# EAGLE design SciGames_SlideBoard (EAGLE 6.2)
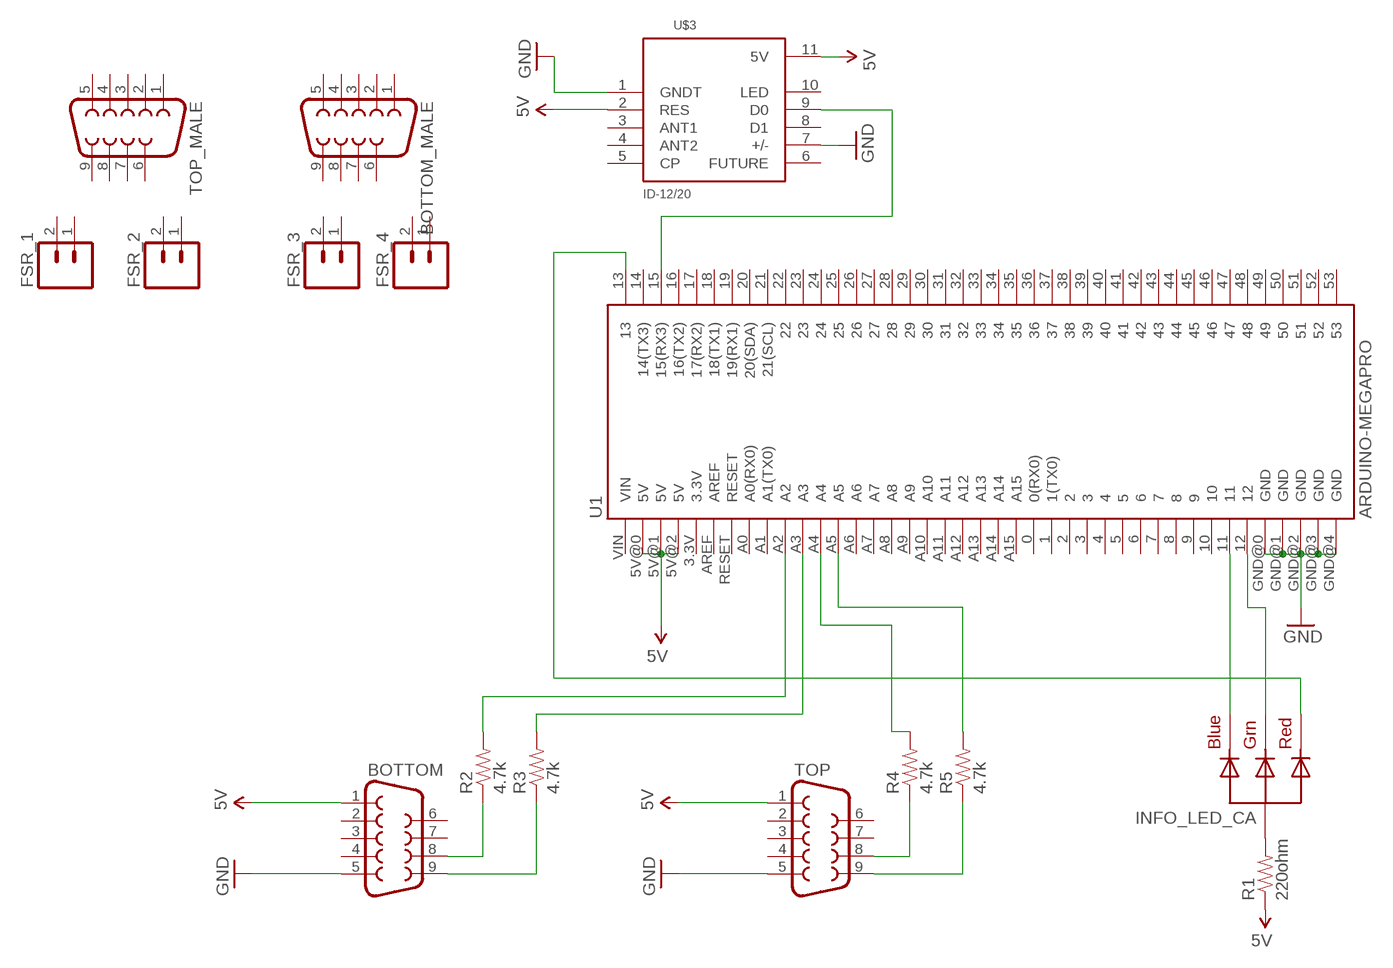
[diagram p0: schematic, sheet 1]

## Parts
BOTTOM  DB9FEMALE  [DB9]
BOTTOM_MALE  DB9MALE  [DB9_MALE]
FSR_1  M02JST-PTH-2  [JST-2-PTH]
FSR_2  M02JST-PTH-2  [JST-2-PTH]
FSR_3  M02JST-PTH-2  [JST-2-PTH]
FSR_4  M02JST-PTH-2  [JST-2-PTH]
INFO_LED_CA  RGBLED_CA-5MM  [LED5MMRGB]
R1  220ohm  RESISTORPTH-1/6W  [1/6W-RES]
R2  4.7k  RESISTORPTH-1/6W  [1/6W-RES]
R3  4.7k  RESISTORPTH-1/6W  [1/6W-RES]
R4  4.7k  RESISTORPTH-1/6W  [1/6W-RES]
R5  4.7k  RESISTORPTH-1/6W  [1/6W-RES]
TOP  DB9FEMALE  [DB9]
TOP_MALE  DB9MALE  [DB9_MALE]
U1  ARDUINO-MEGAPRO  [ARDUINO_MEGA-PRO-3.3V]
U$3  ID-12/20  [ID-12]

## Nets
5V: BOTTOM.1 R1.1 TOP.1 U1.5V@0(5V) U1.5V@1(5V) U1.5V@2(5V) U$3.2(RES) U$3.11(5V)
GND: BOTTOM.5 TOP.5 U1.GND@0(GND) U1.GND@1(GND) U1.GND@2(GND) U1.GND@3(GND) U1.GND@4(GND) U$3.1(GNDT) U$3.7(+/-)
N$1: U1.15(15(RX3)) U$3.9(D0)
N$2: INFO_LED_CA.4(BLUE) U1.11
N$3: INFO_LED_CA.3(GREEN) U1.12
N$4: INFO_LED_CA.1(RED) U1.13
N$5: INFO_LED_CA.2(VCC) R1.2
N$6: BOTTOM.8 R2.1
N$7: BOTTOM.9 R3.1
N$8: R4.1 TOP.8
N$9: R5.1 TOP.9
N$10: R5.2 U1.A5
N$11: R4.2 U1.A4
N$12: R3.2 U1.A3
N$13: R2.2 U1.A2
Unconnected: BOTTOM.2 BOTTOM.3 BOTTOM.4 BOTTOM.6 BOTTOM.7 BOTTOM_MALE.1 BOTTOM_MALE.2 BOTTOM_MALE.3 BOTTOM_MALE.4 BOTTOM_MALE.5 BOTTOM_MALE.6 BOTTOM_MALE.7 BOTTOM_MALE.8 BOTTOM_MALE.9 FSR_1.1 FSR_1.2 FSR_2.1 FSR_2.2 FSR_3.1 FSR_3.2 FSR_4.1 FSR_4.2 TOP.2 TOP.3 TOP.4 TOP.6 TOP.7 TOP_MALE.1 TOP_MALE.2 TOP_MALE.3 TOP_MALE.4 TOP_MALE.5 TOP_MALE.6 TOP_MALE.7 TOP_MALE.8 TOP_MALE.9 U1.0(0(RX0)) U1.1(1(TX0)) U1.2 U1.3 U1.3.3V U1.4 U1.5 U1.6 U1.7 U1.8 U1.9 U1.10 U1.14(14(TX3)) U1.16(16(TX2)) U1.17(17(RX2)) U1.18(18(TX1)) U1.19(19(RX1)) U1.20(20(SDA)) U1.21(21(SCL)) U1.22 U1.23 U1.24 U1.25 U1.26 U1.27 U1.28 U1.29 U1.30 U1.31 U1.32 U1.33 U1.34 U1.35 U1.36 U1.37 U1.38 U1.39 U1.40 U1.41 U1.42 U1.43 U1.44 U1.45 U1.46 U1.47 U1.48 U1.49 U1.50 U1.51 U1.52 U1.53 U1.A0(A0(RX0)) U1.A1(A1(TX0)) U1.A6 U1.A7 U1.A8 U1.A9 U1.A10 U1.A11 U1.A12 U1.A13 U1.A14 U1.A15 U1.AREF U1.RESET U1.VIN U$3.3(ANT1) U$3.4(ANT2) U$3.5(CP) U$3.6(FUTURE) U$3.8(D1) U$3.10(LED)

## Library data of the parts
BOTTOM BOTTOM_MALE TOP TOP_MALE = SparkFun-Connectors:DB9: DB9 Connector Standard DB9 (D-Sub 9) serial connector. Can be used for CAN bus as well as RS485 and RS232. Footprint production proven. Spark Fun Electronics SKU : PRT-00429
FSR_1-FSR_4 = SparkFun-Connectors:M02: Header 2
INFO_LED_CA = adafruit:RGBLED_CA: RGB LED, common-anode 5MM Staggered pins 5mm Piranha package http://www.ladyada.net/library/pcb/eaglelibrary.html
R1-R5 = SparkFun-Passives:RESISTOR: Resistor
U1 = SparkFun:ARDUINO-MEGA: Arduino Mega footprint connections
U$3 = SparkFun-RF:ID-12/20: RFID reader for ID2, ID12, and ID20 Package

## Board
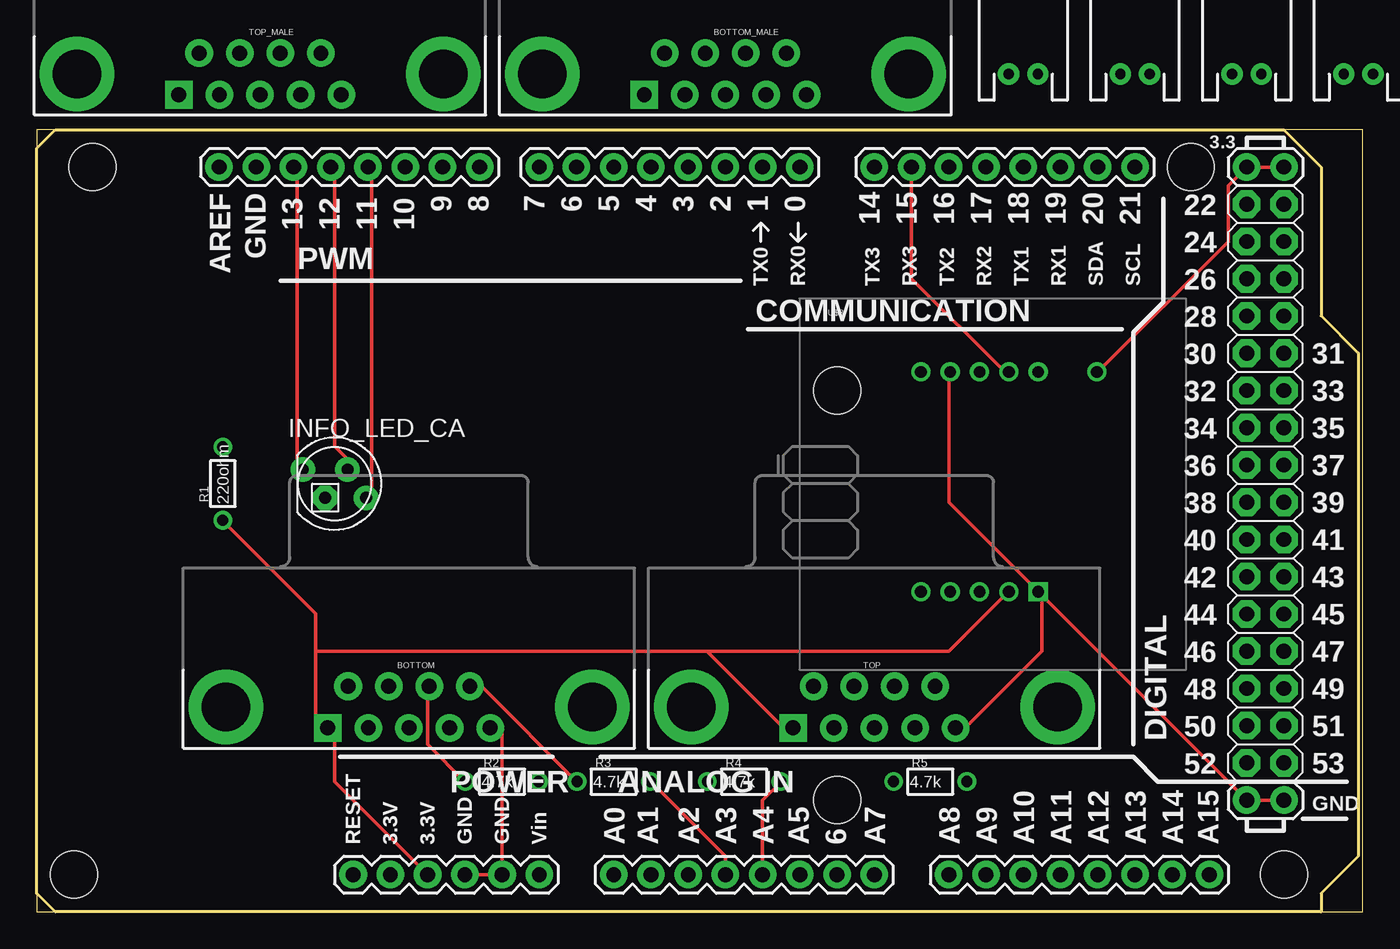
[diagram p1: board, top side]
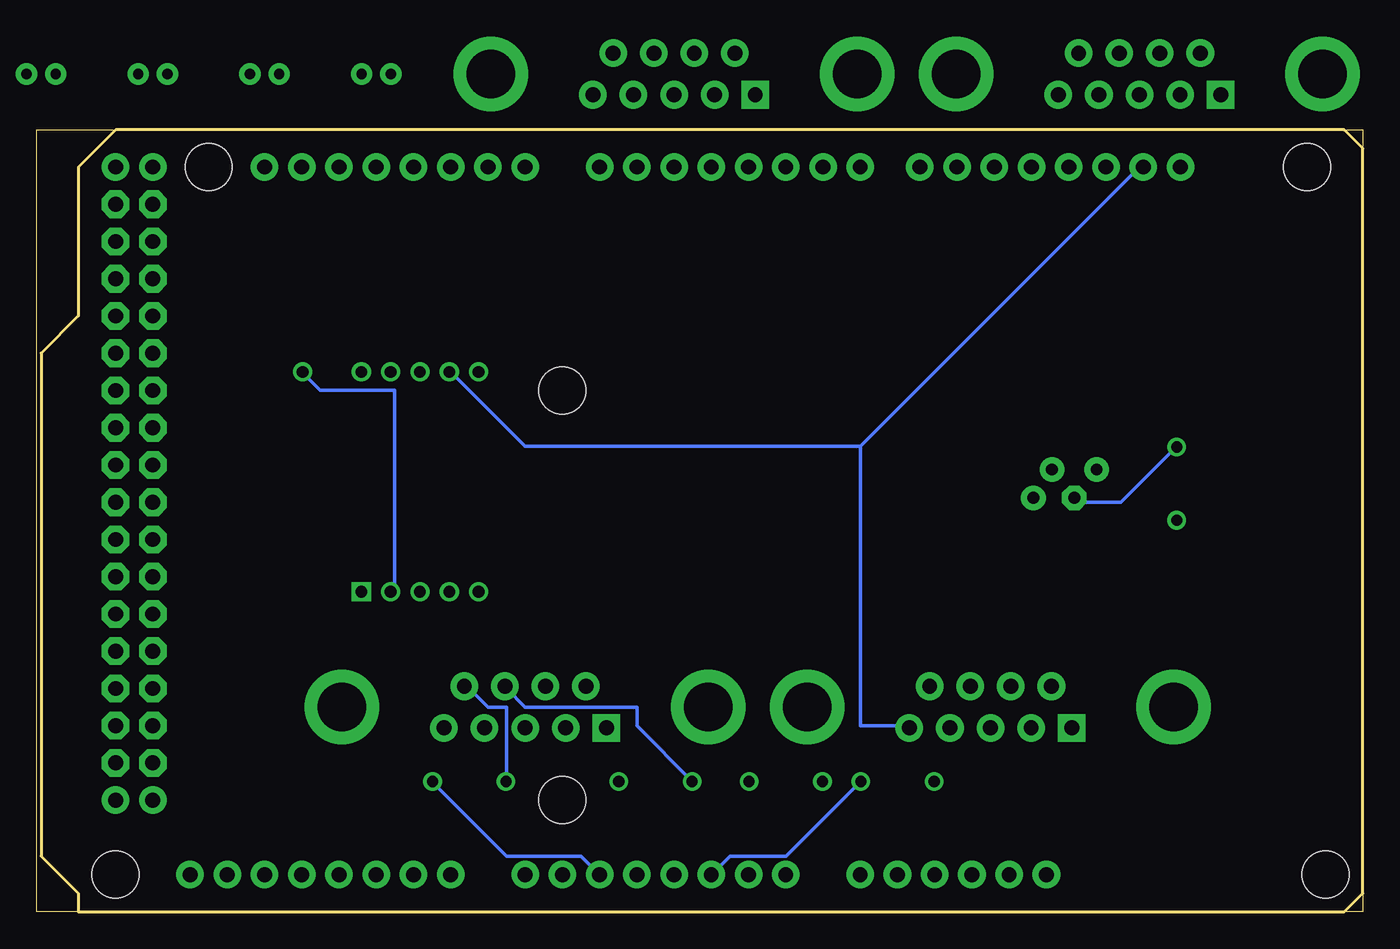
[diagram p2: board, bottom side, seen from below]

Size 90.47 x 53.34 mm. Coordinates in mm from the lower left corner, seen from the top.
Outline: 0,0 90.47,0 90.47,53.33 0,53.33 0,0
Copper layers (1*16): Top 0.035mm / dielectric 1.5mm / Bottom 0.035mm
Design rules: minimum track width 10mil, minimum drill 24mil, track to track 8mil, track to pad 8mil, pad to pad 8mil, via to via 8mil, smd to smd 8mil, copper to edge 40mil, drill to drill 8mil, minimum pad ring 10mil, minimum via ring 8mil, stop-mask expansion 4mil, vias tented up to drill 0mil, thermal gap 10mil

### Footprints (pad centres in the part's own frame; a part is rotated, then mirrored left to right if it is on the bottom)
DB9 = drill 1.016 pad 1.88 square: 1 -5.54,-1.42 | drill 1.016 pad 1.88: 2 -2.77,-1.42; 3 0,-1.42; 4 2.77,-1.42; 5 5.54,-1.42; 6 -4.15,1.42; 7 -1.38,1.42; 8 1.38,1.42; 9 4.15,1.42 | drill 3.302 pad 5.08: G1 -12.5,0; G2 12.5,0
DB9_MALE = drill 1.016 pad 1.88: 1 5.54,-1.42; 2 2.77,-1.42; 3 0,-1.42; 4 -2.77,-1.42; 6 4.15,1.42; 7 1.38,1.42; 8 -1.38,1.42; 9 -4.15,1.42 | drill 1.016 pad 1.88 square: 5 -5.54,-1.42 | drill 3.302 pad 5.08: G1 -12.5,0; G2 12.5,0
JST-2-PTH = drill 0.7 pad 1.448: 1 -1,0; 2 1,0
LED5MMRGB = drill 0.8 pad 1.676: 1 -2.159,0.968; 3 0.889,0.968; 4 2.159,-0.968 | drill 0.8 pad 1.676 octagon: 2 -0.635,-0.968
1/6W-RES = drill 0.762: 1 -2.5,0; 2 2.5,0
ARDUINO_MEGA-PRO-3.3V = drill 1.016 pad 1.88: 0 52.07,50.8; 1 49.53,50.8; 2 46.99,50.8; 3 44.45,50.8; 3.3V 24.13,2.54; 4 41.91,50.8; 5 39.37,50.8; 5V@0 26.67,2.54; 5V@1 82.55,50.8; 5V@2 85.09,50.8; 6 36.83,50.8; 7 34.29,50.8; 8 30.226,50.8; 9 27.686,50.8; 10 25.146,50.8; 11 22.606,50.8; 12 20.066,50.8; 13 17.526,50.8; 14 57.15,50.8; 15 59.69,50.8; 16 62.23,50.8; 17 64.77,50.8; 18 67.31,50.8; 19 69.85,50.8; 20 72.39,50.8; 21 74.93,50.8; A0 39.37,2.54; A1 41.91,2.54; A2 44.45,2.54; A3 46.99,2.54; A4 49.53,2.54; A5 52.07,2.54; A6 54.61,2.54; A7 57.15,2.54; A8 62.23,2.54; A9 64.77,2.54; A10 67.31,2.54; A11 69.85,2.54; A12 72.39,2.54; A13 74.93,2.54; A14 77.47,2.54; A15 80.01,2.54; AREF 12.446,50.8; GND@0 29.21,2.54; GND@1 31.75,2.54; GND@2 82.55,7.62; GND@3 85.09,7.62; GND@4 14.986,50.8; RESET 21.59,2.54; VIN 34.29,2.54 | drill 1.016 pad 1.88 octagon: 22 82.55,48.26; 23 85.09,48.26; 24 82.55,45.72; 25 85.09,45.72; 26 82.55,43.18; 27 85.09,43.18; 28 82.55,40.64; 29 85.09,40.64; 30 82.55,38.1; 31 85.09,38.1; 32 82.55,35.56; 33 85.09,35.56; 34 82.55,33.02; 35 85.09,33.02; 36 82.55,30.48; 37 85.09,30.48; 38 82.55,27.94; 39 85.09,27.94; 40 82.55,25.4; 41 85.09,25.4; 42 82.55,22.86; 43 85.09,22.86; 44 82.55,20.32; 45 85.09,20.32; 46 82.55,17.78; 47 85.09,17.78; 48 82.55,15.24; 49 85.09,15.24; 50 82.55,12.7; 51 85.09,12.7; 52 82.55,10.16; 53 85.09,10.16 | hole 3.2: 3.81,50.8; 2.54,2.54; 54.61,35.56; 54.61,7.62; 78.74,50.8; 85.09,2.54
ID-12 = drill 0.8 square: 1 16.255,5.32 | drill 0.8: 2 14.255,5.32; 3 12.255,5.32; 4 10.255,5.32; 5 8.255,5.32; 6 8.255,20.32; 7 10.255,20.32; 8 12.255,20.32; 9 14.255,20.32; 10 16.255,20.32; 11 20.255,20.32

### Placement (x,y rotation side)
BOTTOM  25.4,13.97 0 top
BOTTOM_MALE  46.99,57.15 0 top
FSR_1  not placed on the board
FSR_2  not placed on the board
FSR_3  not placed on the board
FSR_4  not placed on the board
INFO_LED_CA  20.32,29.21 0 top
R1  12.7,29.21 90 top
R2  31.75,8.89 0 top
R3  39.37,8.89 0 top
R4  48.26,8.89 0 top
R5  60.96,8.89 0 top
TOP  57.15,13.97 0 top
TOP_MALE  15.24,57.15 0 top
U1  0,0 0 top
U$3  52.07,16.51 0 top

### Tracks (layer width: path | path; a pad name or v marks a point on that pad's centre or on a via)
5V
  Top 0.254: U1.5V@2 U1.5V@1 81.28,49.53 81.28,45.72 72.39,36.83 U$3.11 | 19.05,17.78 19.05,12.7 BOTTOM.1 20.32,12.7 20.32,8.89 U1.5V@0 | 19.05,17.78 19.05,20.32 12.7,26.67 R1.1 | 45.72,17.78 50.8,12.7 TOP.1 | 19.05,17.78 45.72,17.78 | 45.72,17.78 62.23,17.78 66.04,21.59 U$3.2
  Bottom 0.254: U$3.2 66.04,21.59 66.04,35.56 71.12,35.56 72.39,36.83 U$3.11
GND
  Top 0.254: U1.GND@0 U1.GND@1 31.75,12.7 BOTTOM.5 | U1.GND@3 U1.GND@2 68.58,21.59 | 68.58,21.59 62.23,27.94 62.23,36.83 U$3.7 | 68.58,21.59 68.58,17.78 63.5,12.7 TOP.5 | 68.58,21.59 U$3.1
  Bottom 0.254: 34.29,31.75 15.24,50.8 U1.GND@4 | 34.29,31.75 34.29,12.7 31.75,12.7 BOTTOM.5 | 34.29,31.75 57.15,31.75 62.23,36.83 U$3.7
N$1
  Top 0.254: U1.15 59.69,43.18 66.04,36.83 U$3.9
N$2
  Top 0.254: INFO_LED_CA.4 22.86,27.94 22.86,50.8 U1.11
N$3
  Top 0.254: INFO_LED_CA.3 21.59,30.48 20.32,31.75 20.32,50.8 U1.12
N$4
  Top 0.254: INFO_LED_CA.1 17.78,30.48 17.78,50.8 U1.13
N$5
  Top 0.254: 20.32,27.94 INFO_LED_CA.2
  Bottom 0.254: R1.2 12.7,31.75 16.51,27.94 19.05,27.94 INFO_LED_CA.2
N$6
  Top 0.254: R2.1 29.21,8.89 26.67,11.43 26.67,15.24 BOTTOM.8
N$7
  Top 0.254: R3.1 36.83,8.89 30.48,15.24 BOTTOM.9
N$8
  Bottom 0.254: R4.1 45.72,8.89 49.53,12.7 49.53,13.97 57.15,13.97 58.42,15.24 TOP.8
N$9
  Bottom 0.254: R5.1 58.42,8.89 58.42,13.97 59.69,13.97 60.96,15.24 TOP.9
N$10
  Bottom 0.254: U1.A5 53.34,3.81 58.42,3.81 63.5,8.89 R5.2
N$11
  Top 0.254: U1.A4 49.53,7.62 50.8,8.89 R4.2
N$12
  Top 0.254: U1.A3 46.99,3.81 41.91,8.89 R3.2
N$13
  Bottom 0.254: U1.A2 43.18,3.81 39.37,3.81 34.29,8.89 R2.2

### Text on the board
tValues: SciGames Slide Board

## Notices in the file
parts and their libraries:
SparkFun: Licensing: CC v3.0 Share-Alike You are welcome to use this library for commercial purposes.
